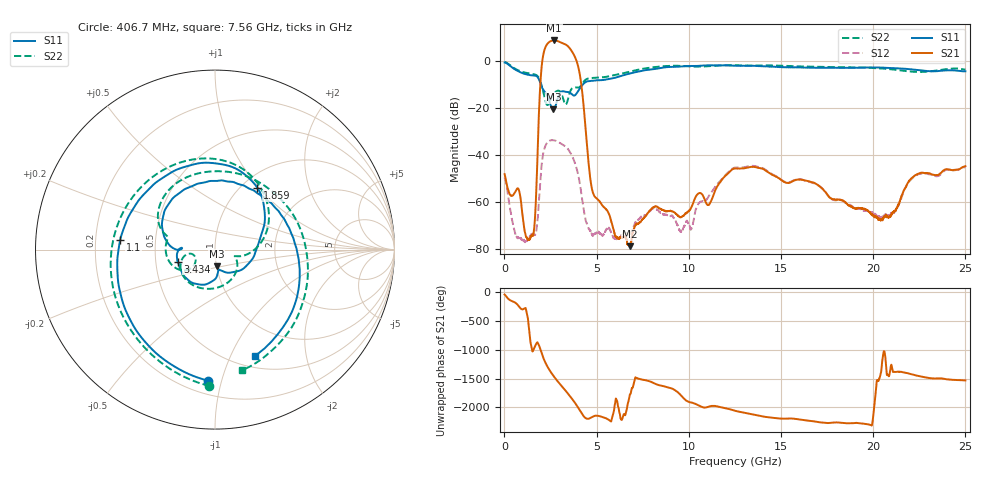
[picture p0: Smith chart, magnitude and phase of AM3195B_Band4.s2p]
!Agilent Technologies,E8364B,MY43040894,A.07.50.67
!Agilent E8364B: A.07.50.67
!Date: Wednesday, July 07, 2021 13:17:55
!Correction: S11(Full 2 Port(1,2))
!S21(Full 2 Port(1,2))
!S12(Full 2 Port(1,2))
!S22(Full 2 Port(1,2))
!S2P File: Measurements: S11, S21, S12, S22:
# Hz S  dB  R 50
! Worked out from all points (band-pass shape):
!   8001 points, 10 MHz to 25 GHz, reference 50 ohm
!   highest |S21| = 8.77 dB at 2.696 GHz (marker M1); lowest = -78.9 dB at 6.795 GHz (marker M2)
!   |S21| within 3 dB of the highest: 2.218 GHz to 3.508 GHz (1.29 GHz wide, 45.1 % of centre)
!   lowest |S11| = -20.6 dB at 2.656 GHz (marker M3), VSWR 1.21, Z = 50.1 - j9.43 ohm
!   |S11| at or under -10 dB: 1.979 GHz to 4.252 GHz (2.273 GHz wide, 72.9 % of centre)
!   |S22| runs from -18.7 to -0.4 dB; largest |S21 - S12| = 2.8
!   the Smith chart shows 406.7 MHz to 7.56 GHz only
!   S11 on the Smith chart (normalised r, x): 406.7 MHz: 0.29, -0.91; 1.1 GHz: 0.31, +0.04; 1.859 GHz: 1.18, +0.98; 3.434 GHz: 0.65, -0.09; 7.56 GHz: 0.63, -1.24
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1e7  -0.63 -11.6  -48.22 -36.9  -49.58 -40.1  -0.40 -12.4
4.067162e8  -2.71 -92.9  -57.48 -150.8  -67.41 -161.0  -2.38 -92.3
1.100189e9  -5.49 174.3  -72.70 82.5  -77.13 31.2  -4.88 174.9
1.85926e9  -7.59 55.4  -24.58 170.2  -61.22 -10.7  -7.13 57.4
2.168511e9  -12.95 -4.0  4.67 -104.9  -37.33 85.9  -15.40 -10.6
2.312204e9  -14.63 -37.4  7.15 160.6  -34.87 -7.3  -18.68 -17.8
2.471515e9  -18.15 -72.2  8.32 74.7  -33.89 -91.5  -16.97 -29.6
2.655816e9  -20.56 -84.2  8.76 -10.8  -33.76 -175.5  -14.00 -71.4
2.696425e9  -20.41 -82.9  8.77 -28.4  -33.80 167.2  -13.64 -81.1
2.865108e9  -16.50 -86.0  8.57 -98.2  -34.24 98.5  -12.71 -117.3
3.061904e9  -13.22 -119.0  7.89 -174.2  -35.19 24.1  -13.49 -155.3
3.43363e9  -13.18 -162.3  6.39 43.2  -37.37 -113.9  -16.70 -143.2
3.714768e9  -14.56 176.9  3.41 -72.6  -41.28 134.9  -11.39 -170.3
4.177082e9  -10.71 165.9  -10.46 60.1  -56.92 -103.4  -10.23 161.0
4.811204e9  -8.40 97.4  -56.36 1.7  -73.89 -93.2  -7.22 95.9
6.794785e9  -5.30 -36.1  -78.92 13.5  -73.74 -116.4  -4.48 -41.0
7.560104e9  -3.99 -69.3  -66.95 -83.5  -65.94 -97.5  -3.23 -77.4
8.341041e9  -3.17 -99.2  -62.48 -169.5  -63.70 -177.0  -2.44 -109.1
1.2505e10  -1.97 141.2  -45.80 100.2  -45.42 100.8  -1.78 127.4
1.667208e10  -2.84 19.0  -51.67 -79.7  -51.82 -82.6  -2.43 3.6
2.083604e10  -2.99 -70.9  -66.69 -17.0  -65.78 -9.3  -3.40 -83.4
2.5e10  -4.37 -119.6  -44.83 -92.2  -45.37 -90.0  -3.67 -130.0
